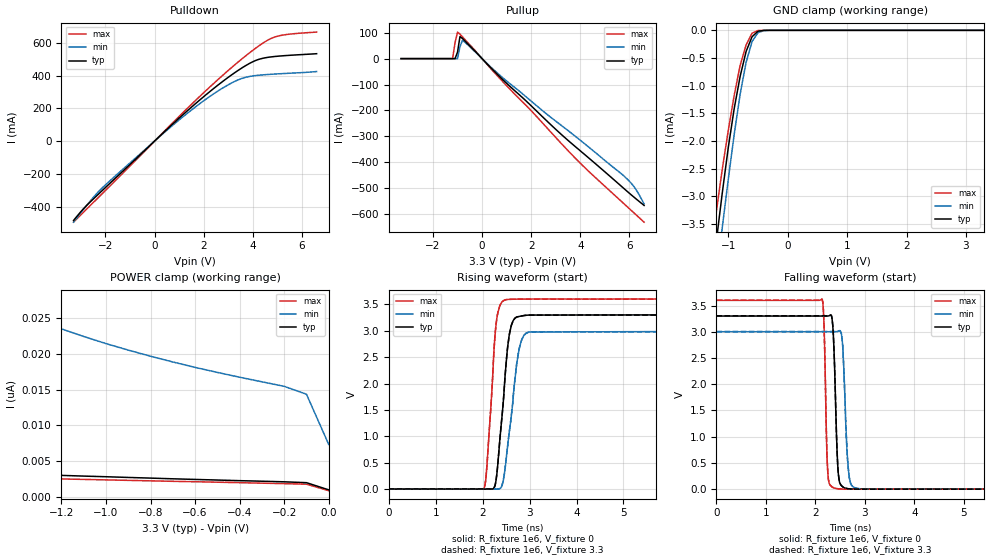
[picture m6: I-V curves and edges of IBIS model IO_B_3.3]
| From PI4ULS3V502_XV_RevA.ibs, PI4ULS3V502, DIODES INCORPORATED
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|   Model IO_B_3.3
[Model]   IO_B_3.3
Model_type  I/O
Vinl=0.99
Vinh=2.31
Enable   Active-High
Vref =   0
|Rref =   1000000
|Cref =   0
Vmeas =   0
| variable   typ   min   max
C_comp   8.864pF   8.757pF   8.982pF
[Driver Schedule]
| Model_Name Rise_on_dly Rise_off_dly Fall_on_dly Fall_off_dly
oneshot_up_B   0ns   1.3ns   NA   NA
oneshot_dw_B   NA   NA   0ns   1.3ns
1K_33   0ns   NA   0ns   NA
[Voltage Range]   3.30V   3.00V   3.60V
[POWER Clamp Reference]   3.30V   3.00V   3.60V
[GND Clamp Reference]   0.00V   0.00V   0.00V
[Temperature Range]   25   85   -40
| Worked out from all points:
|   slope of the pulldown table from 0 to 0.495 V, typ, clamps not added: 7.05 ohm
|   slope of the pullup table from 0 to 0.495 V, typ, clamps not added: 10.2 ohm
|   GND clamp passes 1 mA (typ) near -0.83 V on its own axis
|   rising waveform, R_fixture 1e6, V_fixture 0: 20-80 % time 186ps typ, 225ps min, 150ps max; typ from 0 V to 3.31 V
|   falling waveform, R_fixture 1e6, V_fixture 0: 20-80 % time 64.4ps typ, 78.7ps min, 50.3ps max; typ from 3.3 V to 0 V
|   rising waveform, R_fixture 1e6, V_fixture 3.3: 20-80 % time 185ps typ, 223ps min, 149ps max; typ from 0.004 V to 3.3 V
|   falling waveform, R_fixture 1e6, V_fixture 3.3: 20-80 % time 64.4ps typ, 78.7ps min, 50.4ps max; typ from 3.3 V to 0 V
[GND Clamp]
| Voltage   I(typ)   I(min)   I(max)
-3.3V     -24.17mA   -24.42mA   -24.09mA
-1.3V     -4.71mA    -5.353mA   -4.125mA
-1.2V     -3.802mA   -4.445mA   -3.269mA
-1.1V     -2.929mA   -3.554mA   -2.501mA
-1V       -2.118mA   -2.692mA   -1.809mA
-900mV    -1.411mA   -1.878mA   -1.173mA
-800mV    -829.8uA   -1.151mA   -632.5uA
-700mV    -381.7uA   -576.7uA   -263uA
-600mV    -116.2uA   -203.6uA   -52.63uA
-500mV    -16.3uA    -42uA      -3.416uA
-400mV    -1.145uA   -5.033uA   -91.97nA
3.3V      1.01nA     16.27nA    23.98pA
[POWER Clamp]
| Voltage   I(typ)   I(min)   I(max)
-3.3V     6.818nA    89.17nA    3.932nA
-3V       5.933nA    71.31nA    3.74nA
-2.5V     4.813nA    49.93nA    3.389nA
-1.6V     3.476nA    28.72nA    2.808nA
-1.5V     3.356nA    27.24nA    2.739nA
-1.3V     3.13nA     24.63nA    2.602nA
-1V       2.842nA    21.42nA    2.402nA
-800mV    2.65nA     19.66nA    2.268nA
-600mV    2.465nA    18.1nA     2.143nA
-200mV    2.132nA    15.46nA    1.877nA
-100mV    2.012nA    14.35nA    1.799nA
0V        1.01nA     7.337nA    893.5pA
[Pulldown]
| Voltage   I(typ)   I(min)   I(max)
-3.3V     -484.4mA   -494.4mA   -495mA
-2.9V     -413.8mA   -418mA     -435.4mA
-2.4V     -340mA     -327.5mA   -360.8mA
-1.8V     -254.9mA   -239.9mA   -271.6mA
1V        139.9mA    129mA      150.7mA
1.9V      258.3mA    234.8mA    281mA
2.7V      355.3mA    316.8mA    391.2mA
3.6V      450.3mA    384.4mA    506.6mA
4.2V      496.5mA    401.2mA    575.9mA
4.7V      512.8mA    407.3mA    623mA
5.3V      521.4mA    412.5mA    648.7mA
6.6V      533.2mA    424.3mA    665.2mA
[Pullup]
| Voltage   I(typ)   I(min)   I(max)
-3.3V     7.384nA    106.3nA    698.3pA
-1.2V     1.902nA    30.02nA    373pA
-1.1V     1.792nA    28.45nA    61.69mA
-1V       24.84mA    27.01nA    102.3mA
-900mV    85.13mA    45.8mA     94.03mA
-800mV    77.63mA    70.59mA    84.05mA
-700mV    68.37mA    63.38mA    73.81mA
900mV     -86.21mA   -78.38mA   -94.49mA
3.7V      -331.6mA   -292.2mA   -374.6mA
5.8V      -502.9mA   -454.6mA   -561.6mA
6.2V      -535.4mA   -495.5mA   -596.3mA
6.6V      -566.5mA   -560.7mA   -631mA
[Rising Waveform]
| IO_33
R_fixture =   1e6
C_fixture =   0
L_fixture =   0
V_fixture =   0
V_fixture_min = 0
V_fixture_max = 0
|   Time   V(typ)   V(min)   V(max)
0s        228.7uV    317.7uV    166.8uV
2.025ns   218.9uV    284.3uV    14.09mV
2.087ns   190.8uV    289.3uV    407mV
2.275ns   118.8mV    -474.4uV   3.04V
2.462ns   1.948V     289.4mV    3.58V
2.525ns   2.639V     766.2mV    3.593V
2.612ns   3.107V     1.404V     3.597V
2.775ns   3.271V     2.651V     3.6V
2.975ns   3.297V     2.972V     3.601V
12ns      3.308V     2.999V     3.601V
[Falling Waveform]
| IO_33
R_fixture =   1e6
C_fixture =   0
L_fixture =   0
V_fixture =   0
V_fixture_min = 0
V_fixture_max = 0
|   Time   V(typ)   V(min)   V(max)
0s        3.299V     3.001V     3.598V
2.137ns   3.299V     3V         3.616V
2.175ns   3.299V     3V         3.102V
2.25ns    3.3V       3.001V     320.1mV
2.387ns   2.34V      3V         20.24mV
2.487ns   132.4mV    3.018V     5.045mV
2.55ns    46.78mV    2.75V      2.167mV
2.675ns   7.287mV    291.3mV    651.4uV
2.812ns   1.294mV    21.91mV    302.6uV
12ns      320uV      2.136mV    1.198mV
[Rising Waveform]
| IO_33
R_fixture =   1e6
C_fixture =   0
L_fixture =   0
V_fixture =   3.3
V_fixture_min = 3
V_fixture_max = 3.6
|   Time   V(typ)   V(min)   V(max)
0s        4.049mV    3.94mV     4.232mV
2.025ns   4.041mV    3.909mV    18.14mV
2.087ns   4.012mV    3.914mV    409.3mV
2.275ns   122mV      3.144mV    3.04V
2.462ns   1.948V     291.8mV    3.58V
2.525ns   2.639V     767.7mV    3.593V
2.612ns   3.108V     1.405V     3.597V
2.775ns   3.271V     2.651V     3.6V
2.975ns   3.297V     2.972V     3.601V
12ns      3.298V     2.978V     3.601V
[Falling Waveform]
| IO_33
R_fixture =   1e6
C_fixture =   0
L_fixture =   0
V_fixture =   3.3
V_fixture_min = 3
V_fixture_max = 3.6
|   Time   V(typ)   V(min)   V(max)
0s        3.304V     3.005V     3.603V
2.137ns   3.304V     3.005V     3.62V
2.175ns   3.303V     3.005V     3.107V
2.25ns    3.304V     3.005V     321.5mV
2.387ns   2.344V     3.004V     20.3mV
2.487ns   132.7mV    3.022V     5.077mV
2.55ns    46.91mV    2.755V     2.196mV
2.675ns   7.32mV     292.4mV    673.1uV
2.812ns   1.321mV    21.99mV    326uV
12ns      244.1uV    2.164mV    1.368mV
[Ramp]
| variable   typ   min   max
dV/dt_r   1.98/187.4E-12   1.80/214.7E-12   2.16/151.6E-12
dV/dt_f   1.98/66.3E-12   1.80/75.0E-12   2.16/51.5E-12
R_load = 1.00E+6
